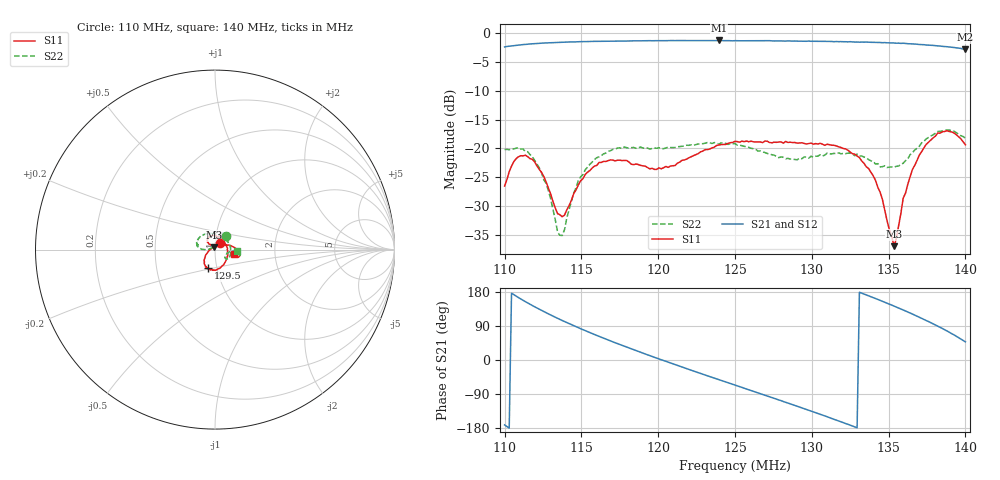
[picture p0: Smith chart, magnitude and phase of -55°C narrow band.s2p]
!Agilent Technologies,E8362C,SG49020144,A.09.33.09
!Agilent E8362C: A.09.33.09
!Date: Friday, October 10, 2025 08:56:21
!Correction: S11(Full 2 Port(1,2))
!S21(Full 2 Port(1,2))
!S12(Full 2 Port(1,2))
!S22(Full 2 Port(1,2))
!S2P File: Measurements: S11, S21, S12, S22:
# Hz S  dB  R 50
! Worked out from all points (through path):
!   201 points, 110 MHz to 140 MHz, reference 50 ohm
!   highest |S21| = -1.26 dB at 124 MHz (marker M1); lowest = -2.8 dB at 140 MHz (marker M2)
!   lowest |S11| = -37.0 dB at 135.3 MHz (marker M3), VSWR 1.03, Z = 49.4 + j1.28 ohm
!   |S11| at or under -10 dB: start of sweep to end of sweep
!   |S22| runs from -35.1 to -16.8 dB; largest |S21 - S12| = 0.0072
!   S11 on the Smith chart (normalised r, x): 110 MHz: 1.05, +0.08; 129.5 MHz: 0.91, -0.19; 140 MHz: 1.23, -0.07
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1.1e8  -26.53 56.4  -2.39 -171.3  -2.40 -171.3  -20.19 51.7
1.106e8  -22.28 72.0  -2.15 172.3  -2.17 172.4  -20.09 67.8
1.1135e8  -21.18 65.0  -1.96 154.0  -1.95 154.1  -20.55 69.0
1.127e8  -25.82 56.4  -1.69 124.8  -1.70 124.8  -26.06 65.1
1.136e8  -31.50 85.4  -1.58 107.1  -1.59 107.1  -35.08 105.4
1.151e8  -25.26 133.2  -1.45 80.0  -1.46 80.1  -24.56 179.9
1.175e8  -22.04 97.5  -1.37 40.9  -1.35 40.9  -19.90 168.1
1.2005e8  -23.37 21.7  -1.30 2.8  -1.34 2.8  -19.88 164.7
1.2185e8  -21.85 -34.2  -1.28 -22.9  -1.30 -22.9  -19.45 163.1
1.2395e8  -19.40 -74.8  -1.26 -51.8  -1.33 -51.9  -19.27 149.6
1.25e8  -18.76 -87.9  -1.29 -66.2  -1.31 -66.3  -19.17 136.8
1.2725e8  -18.97 -104.8  -1.30 -97.1  -1.31 -97.1  -20.96 94.8
1.295e8  -19.14 -109.7  -1.38 -128.4  -1.39 -128.5  -21.49 32.9
1.301e8  -19.25 -112.8  -1.41 -136.9  -1.43 -137.0  -21.53 16.7
1.331e8  -21.60 -136.8  -1.56 178.7  -1.53 178.7  -21.30 -36.5
1.3415e8  -25.55 -152.7  -1.58 162.3  -1.61 162.2  -22.72 -38.0
1.3505e8  -34.12 161.5  -1.67 147.4  -1.68 147.4  -23.23 -29.2
1.3535e8  -36.97 114.3  -1.70 142.2  -1.71 142.2  -23.28 -23.7
1.3595e8  -28.63 49.9  -1.74 132.0  -1.80 131.9  -22.58 -12.4
1.3745e8  -19.30 6.7  -2.05 104.1  -2.05 104.3  -18.34 -5.3
1.388e8  -16.92 -14.1  -2.35 76.6  -2.36 76.5  -16.81 -11.7
1.4e8  -19.37 -14.6  -2.79 47.9  -2.79 48.0  -18.22 -2.9
